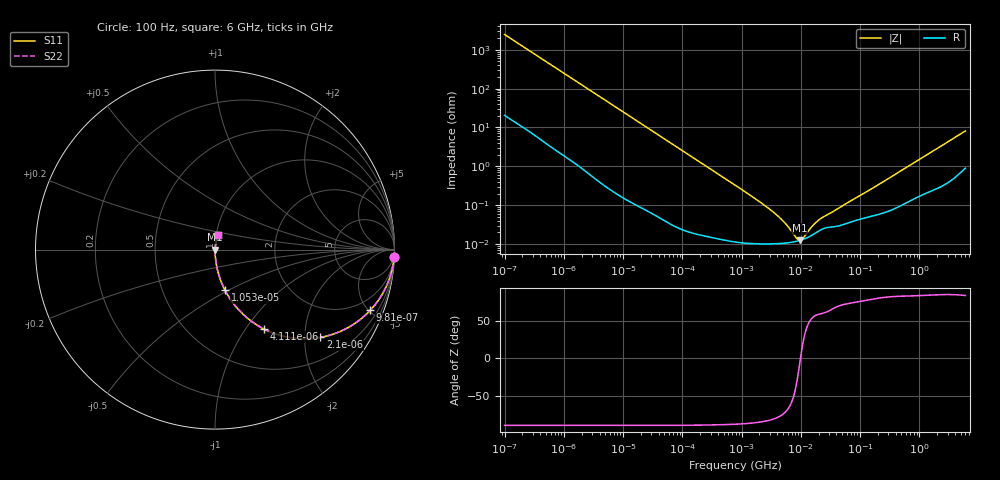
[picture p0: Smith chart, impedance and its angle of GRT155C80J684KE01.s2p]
!Murata Part Number: GRT155C80J684KE01
!These Parameters are Measured in Series Mode Connection
!Data Generated on Jun 19, 2026
!  o--ll--o
!Port1  Port2
!  o------o
!Operation Temp=25[degC], DC Bias Voltage=0[V]
!Freq. Start=100[Hz] Stop=6[GHz] 401[Steps]
# Hz S RI R 50
!Freq.(Hz) S11(Real) S11(Imag) S21(Real) S21(Imag) S12(Real) S12(Imag) S22(Real) S22(Imag)
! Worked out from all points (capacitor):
!   401 points, 100 Hz to 6 GHz, reference 50 ohm
!   read as one part in series: C = 643 nF near 109 Hz
!   lowest |Z| = 12.5 mohm at 9.506 MHz (marker M1)
!   series resonance near 9.874 MHz, so ESL is about 400 pH
!   S11 on the Smith chart (normalised r, x): 100 Hz: 1, -49; 981 Hz: 1.04, -5.09; 2.1 kHz: 1.02, -2.39; 4.111 kHz: 1.01, -1.22; 10.53 kHz: 1.00, -0.48; 6 GHz: 1.02, +0.16
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100  0.998 -0.0404  0.00197 0.0404  0.00197 0.0404  0.998 -0.0404
335  0.9811 -0.132  0.0189 0.132  0.0189 0.132  0.9811 -0.132
600  0.9438 -0.2265  0.0562 0.2265  0.0562 0.2265  0.9438 -0.2265
981  0.8646 -0.3384  0.1354 0.3384  0.1354 0.3384  0.8646 -0.3384
2008  0.6086 -0.4845  0.3914 0.4845  0.3914 0.4845  0.6086 -0.4845
2100  0.5873 -0.4888  0.4127 0.4888  0.4127 0.4888  0.5873 -0.4888
2873  0.4337 -0.4923  0.5663 0.4923  0.5663 0.4923  0.4337 -0.4923
4111  0.2737 -0.4427  0.7263 0.4427  0.7263 0.4427  0.2737 -0.4427
6433  0.1344 -0.3381  0.8656 0.3381  0.8656 0.3381  0.1344 -0.3381
10527  0.0556 -0.226  0.9444 0.226  0.9444 0.226  0.0556 -0.226
19704  0.017 -0.126  0.983 0.126  0.983 0.126  0.017 -0.126
40335  0.00441 -0.0626  0.9956 0.0626  0.9956 0.0626  0.00441 -0.0626
774597  0.000124 -0.00329  0.9999 0.00329  0.9999 0.00329  0.000124 -0.00329
3712478  0.000102 -0.000594  0.9999 0.000594  0.9999 0.000594  0.000102 -0.000594
5554849  0.000106 -0.000315  0.9999 0.000315  0.9999 0.000315  0.000106 -0.000315
8311524  0.000117 -8.92e-05  0.9999 8.92e-05  0.9999 8.92e-05  0.000117 -8.92e-05
9506416  0.000123 -1.94e-05  0.9999 1.94e-05  0.9999 1.94e-05  0.000123 -1.94e-05
1.087309e7  0.000132 4.94e-05  0.9999 -4.94e-05  0.9999 -4.94e-05  0.000132 4.94e-05
1.555665e7  0.00017 0.000232  0.9998 -0.000232  0.9998 -0.000232  0.00017 0.000232
2.327686e7  0.000244 0.00042  0.9998 -0.00042  0.9998 -0.00042  0.000244 0.00042
3.124326e8  0.000739 0.00497  0.9993 -0.00497  0.9993 -0.00497  0.000739 0.00497
6e9  0.0152 0.0788  0.9848 -0.0788  0.9848 -0.0788  0.0152 0.0788
